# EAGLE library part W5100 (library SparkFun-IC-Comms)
WIZnet W5100 TCP/IP PHY Embedded Chip Package: LQFP-80,10x10mm, 0.4mm pitch Note: There is no internal production part or ID for this IC. Datasheet SparkFun Products WIZnet W5100 Network Module with Mag Jack - WIZ811MJ (DEV-09473)
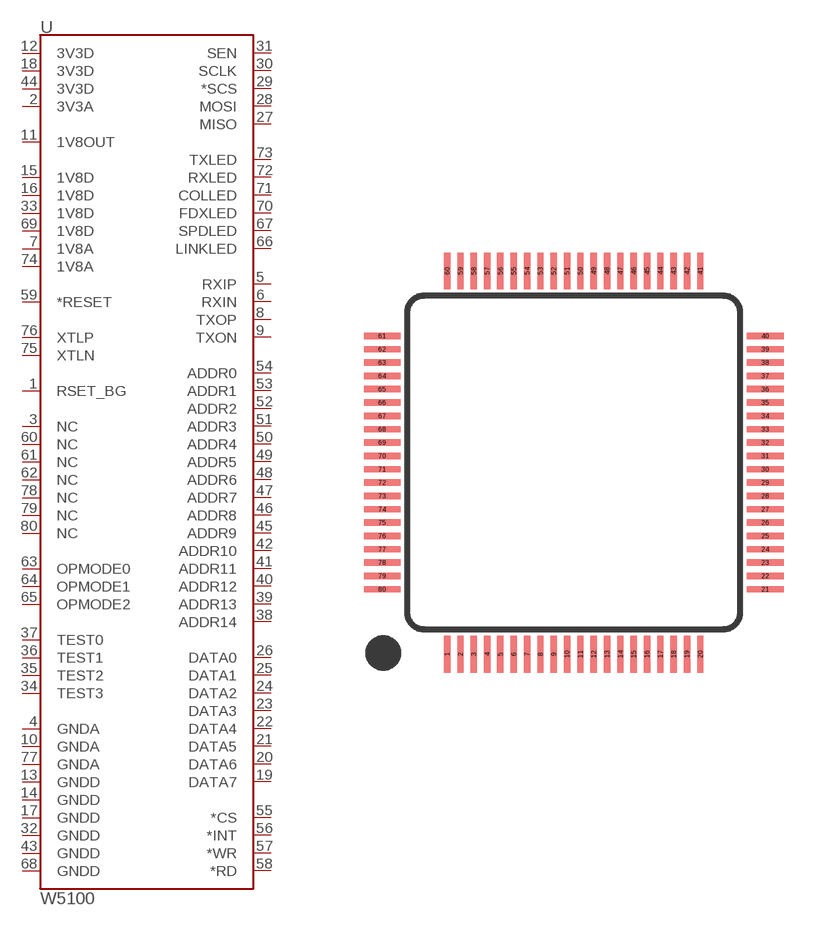
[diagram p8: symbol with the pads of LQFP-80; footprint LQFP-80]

Designator prefix U

## W5100 (PROD_ID: NA-XXXXX; VALUE: W5100)  [LQFP-80]
1  RSET_BG
2  3V3A
3  NC
4  GNDA
5  RXIP
6  RXIN
7  1V8A
8  TXOP
9  TXON
10  GNDA
11  1V8OUT
12  3V3D
13  GNDD
14  GNDD
15  1V8D
16  1V8D
17  GNDD
18  3V3D
19  DATA7
20  DATA6
21  DATA5
22  DATA4
23  DATA3
24  DATA2
25  DATA1
26  DATA0
27  MISO
28  MOSI
29  *SCS
30  SCLK
31  SEN
32  GNDD
33  1V8D
34  TEST3
35  TEST2
36  TEST1
37  TEST0
38  ADDR14
39  ADDR13
40  ADDR12
41  ADDR11
42  ADDR10
43  GNDD
44  3V3D
45  ADDR9
46  ADDR8
47  ADDR7
48  ADDR6
49  ADDR5
50  ADDR4
51  ADDR3
52  ADDR2
53  ADDR1
54  ADDR0
55  *CS
56  *INT
57  *WR
58  *RD
59  *RESET
60  NC
61  NC
62  NC
63  OPMODE0
64  OPMODE1
65  OPMODE2
66  LINKLED
67  SPDLED
68  GNDD
69  1V8D
70  FDXLED
71  COLLED
72  RXLED
73  TXLED
74  1V8A
75  XTLN
76  XTLP
77  GNDA
78  NC
79  NC
80  NC

## Footprint LQFP-80 (pad centres in mm)
LQFP-80 80-pin, 10x10mm, 0.4mm pitch, SMD package Used for WIZnet W5100 (COM-09471) http://www.sparkfun.com/products/9471
smd 0.19 x 1.1: 1 -3.8,-5.75; 2 -3.4,-5.75; 3 -3,-5.75; 4 -2.6,-5.75; 5 -2.2,-5.75; 6 -1.8,-5.75; 7 -1.4,-5.75; 8 -1,-5.75; 9 -0.6,-5.75; 10 -0.2,-5.75; 11 0.2,-5.75; 12 0.6,-5.75; 13 1,-5.75; 14 1.4,-5.75; 15 1.8,-5.75; 16 2.2,-5.75; 17 2.6,-5.75; 18 3,-5.75; 19 3.4,-5.75; 20 3.8,-5.75; 41 3.8,5.75; 42 3.4,5.75; 43 3,5.75; 44 2.6,5.75; 45 2.2,5.75; 46 1.8,5.75; 47 1.4,5.75; 48 1,5.75; 49 0.6,5.75; 50 0.2,5.75; 51 -0.2,5.75; 52 -0.6,5.75; 53 -1,5.75; 54 -1.4,5.75; 55 -1.8,5.75; 56 -2.2,5.75; 57 -2.6,5.75; 58 -3,5.75; 59 -3.4,5.75; 60 -3.8,5.75
smd 1.1 x 0.19: 21 5.75,-3.8; 22 5.75,-3.4; 23 5.75,-3; 24 5.75,-2.6; 25 5.75,-2.2; 26 5.75,-1.8; 27 5.75,-1.4; 28 5.75,-1; 29 5.75,-0.6; 30 5.75,-0.2; 31 5.75,0.2; 32 5.75,0.6; 33 5.75,1; 34 5.75,1.4; 35 5.75,1.8; 36 5.75,2.2; 37 5.75,2.6; 38 5.75,3; 39 5.75,3.4; 40 5.75,3.8; 61 -5.75,3.8; 62 -5.75,3.4; 63 -5.75,3; 64 -5.75,2.6; 65 -5.75,2.2; 66 -5.75,1.8; 67 -5.75,1.4; 68 -5.75,1; 69 -5.75,0.6; 70 -5.75,0.2; 71 -5.75,-0.2; 72 -5.75,-0.6; 73 -5.75,-1; 74 -5.75,-1.4; 75 -5.75,-1.8; 76 -5.75,-2.2; 77 -5.75,-2.6; 78 -5.75,-3; 79 -5.75,-3.4; 80 -5.75,-3.8

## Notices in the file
Licensing: Creative Commons ShareAlike 4.0 International - https://creativecommons.org/licenses/by-sa/4.0
